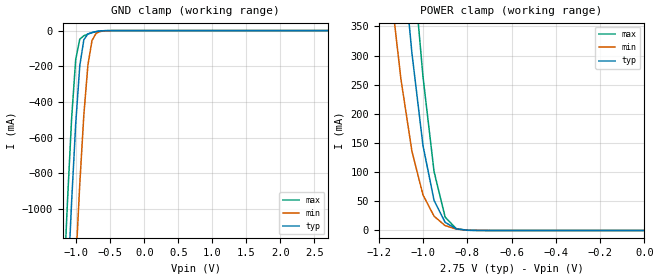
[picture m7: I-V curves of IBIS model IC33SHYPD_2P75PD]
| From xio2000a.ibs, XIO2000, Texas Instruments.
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|   Model IC33SHYPD_2P75PD
[Model]   IC33SHYPD_2P75PD
Model_type   Input
Polarity   Non-Inverting
Vinh =   1.93V
Vinl =   0.82V
|   typ   min   max
C_comp   1.68pF   1.68pF   1.68pF
[Model Spec]
|   typ   min   max
Vinh   1.930V   1.750V   2.10V
Vinl   0.820V   0.750V   0.90V
[Temperature Range]   25.0000   0.1250k   -40.0000
[Voltage Range]   2.7500V   2.5000V   3.0000V
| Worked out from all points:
|   GND clamp passes 1 mA (typ) near -0.60 V on its own axis
|   POWER clamp passes 1 mA (typ) near -0.81 V on its own axis
| (Vdd votage range)   1.50V   1.35V   1.65V
[GND_clamp]
| voltage   I(typ)   I(min)   I(max)
-2.75V    -17.02A    -17.82A    -16.57A
-1.19V    -1.973A    -2.848A    -1.462A
-1.13V    -1.453A    -2.319A    -952.1mA
-1.07V    -961.9mA   -1.806A    -494.2mA
-1.01V    -524.5mA   -1.315A    -162.9mA
-950mV    -197.8mA   -862.4mA   -48.44mA
-890mV    -51.23mA   -472.9mA   -28.95mA
-830mV    -18.97mA   -192.8mA   -19.47mA
-770mV    -10.44mA   -56.15mA   -11.77mA
-710mV    -5.644mA   -15.31mA   -5.841mA
-650mV    -2.514mA   -5.088mA   -2.147mA
2.71V     156.7pA    2.543nA    138.8pA
[POWER_clamp]
| voltage   I(typ)   I(min)   I(max)
-2.75V    9.52A      8.729A     10.16A
-1.15V    732.8mA    427.8mA    979.7mA
-1.1V     506.2mA    260.6mA    722.8mA
-1.05V    304.3mA    136mA      480.1mA
-1V       145.5mA    61.04mA    263.8mA
-950mV    51.56mA    24.44mA    101mA
-900mV    14.01mA    8.383mA    22.94mA
-850mV    2.793mA    2.36mA     3.142mA
-800mV    442.5uA    587.5uA    300.2uA
-750mV    66.2uA     140.7uA    26.86uA
0V        160.3pA    2.35nA     156pA
